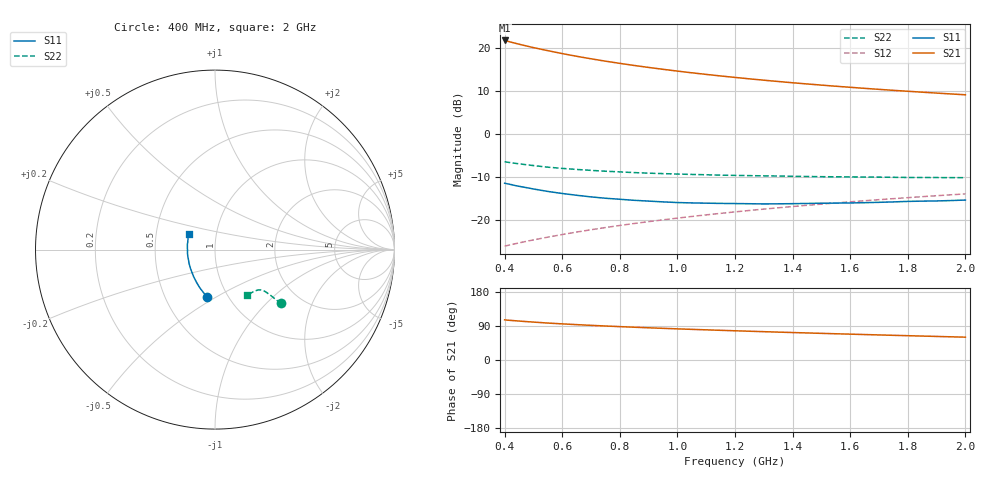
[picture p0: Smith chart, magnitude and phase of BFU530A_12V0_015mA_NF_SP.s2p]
! Filename:  P:\Prog\Test\Noise\ATS_data\Testdata_Net\06 Compressed Noise after Statistics\BFU530A_APG2013_33_A05_12p0V_015mA_NF_CM01_D.sf
! Date/Time: Tue 16/Apr/2013 15:11:00
! BFU530A_APG2013_33_A05_12p0V_1to25mA_NF_CM01_Bias6_R.sf
! Noise Parameter Data File
! BFU530A_APG2013_33_A05_12p0V_1to25mA_NF_CM01
! Date/time: Fri Apr 12 17:55:00 2013
! VAR V_out= 12.001000
! VAR I_out= 15.000000
! VAR V_in= 0.797600
! VAR I_in= 0.140200
! Device data file deembeded for feedlines and parallel
! Original file: \06 Compressed Noise after Statistics\BFU530A_APG2013_33_A05_12p0V_015mA_NF_CM01_R.sf
! Feed-files: PR017V01_150413_Feed1.s2p, PR017V01_150413_Feed2.s2p
! Parallel-file: PR017V01_150413_Par.s2p
# MHz S MA R 50
!  Freq-MHz  S11-mag  S11-arg  S21-mag  S21-arg  S12-mag  S12-arg  S22-mag  S22-arg
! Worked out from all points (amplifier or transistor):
!   37 points, 400 MHz to 2 GHz, reference 50 ohm
!   highest |S21| = 21.8 dB at 400 MHz (marker M1)
!   |S21| within 3 dB of that: start of sweep to 595.4 MHz
!   unconditionally stable (mu >= 1): 1.203 GHz to end of sweep
!   at 500 MHz: K = 0.87, MSG = 22.4 dB, |S12| = -24.7 dB
!   at 1.1 GHz: K = 0.99, MSG = 16.4 dB, |S12| = -18.9 dB
!   at 2 GHz: K = 1.00, MAG = 11.1 dB, |S12| = -14.0 dB
!   lowest NFmin = 0.95 dB at 460 MHz
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400  0.2669 -99.2  12.37 105.9  0.04923 68.2  0.4758 -39.0
420  0.2586 -101.8  11.88 104.6  0.05106 68.4  0.4646 -39.2
440  0.2496 -104.5  11.42 103.3  0.05284 68.5  0.4548 -39.2
460  0.2425 -106.7  10.98 102.2  0.05464 68.7  0.446 -39.4
480  0.2357 -109.2  10.59 101.1  0.05646 68.8  0.437 -39.4
500  0.2289 -111.6  10.22 100.0  0.05825 69.0  0.4294 -39.4
550  0.2142 -117.3  9.408 97.5  0.0627 69.3  0.411 -39.4
600  0.2027 -122.4  8.696 95.3  0.0673 69.6  0.3979 -39.5
650  0.1933 -127.5  8.089 93.3  0.07193 69.9  0.3868 -39.6
700  0.185 -132.3  7.56 91.4  0.07652 70.1  0.3773 -39.7
750  0.1784 -136.9  7.093 89.7  0.08118 70.3  0.3688 -39.8
800  0.1736 -141.2  6.686 88.1  0.08584 70.3  0.3622 -40.0
850  0.1688 -145.8  6.32 86.5  0.09049 70.4  0.3554 -40.3
950  0.1618 -154.0  5.699 83.6  0.09988 70.4  0.3459 -40.9
1050  0.1573 -161.4  5.189 80.9  0.1094 70.3  0.3382 -41.6
1100  0.1563 -165.1  4.969 79.6  0.1141 70.2  0.3353 -42.0
1200  0.1547 -171.8  4.583 77.1  0.1237 69.9  0.3297 -43.0
1350  0.1536 178.9  4.108 73.6  0.138 69.3  0.3239 -44.8
1500  0.1561 170.4  3.728 70.3  0.1524 68.6  0.3185 -46.8
1650  0.1584 163.2  3.417 67.2  0.1669 67.8  0.3154 -49.1
1750  0.1616 158.7  3.239 65.1  0.1765 67.2  0.3131 -50.6
2000  0.17 148.8  2.875 60.3  0.2005 65.5  0.3099 -55.0
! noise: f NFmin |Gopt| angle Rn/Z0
400  0.9728  0.1222  -173.8  0.1004
460  0.9538  0.1435  -172.8  0.0893
600  1.053  0.1255  -159  0.1101
800  1.031  0.1458  -162.9  0.0934
1000  1.044  0.1632  -158.4  0.0924
1200  1.093  0.1697  -154  0.0961
1400  1.106  0.2011  -149.3  0.0945
1600  1.105  0.2099  -142.9  0.1012
1800  1.083  0.2325  -138.7  0.103
2000  1.112  0.2674  -135.2  0.0977
